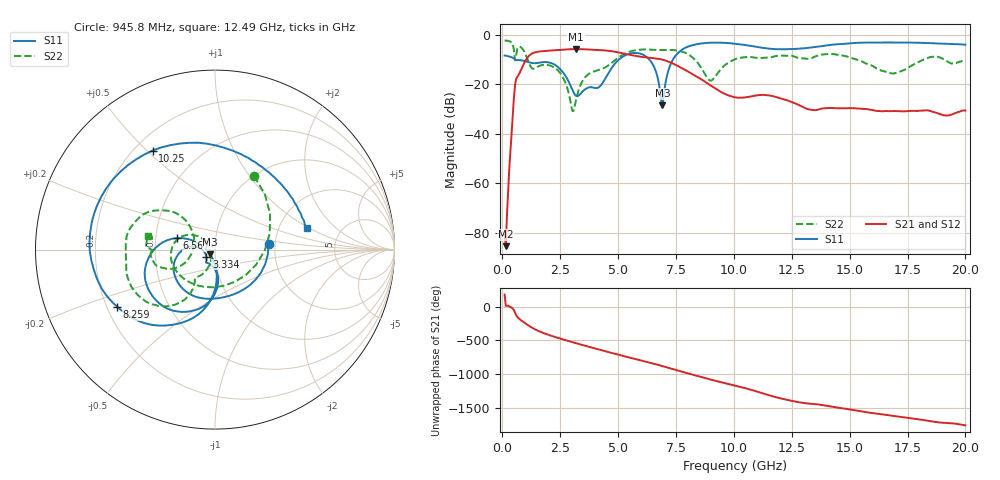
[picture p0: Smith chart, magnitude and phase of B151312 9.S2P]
!  2-Port S-parameters saved by WinCal
! VAR MeasName=S-Parameters (CALIBRATED_DATA) read from VNA (N5244A)
! VAR MeasDate=12/8/2015 5:44:21 PM
! VAR NAME=B151312 9
! VAR FILENAME=B151312 9.S2P
! VAR DATE=12/8/2015 5:44:21 PM
! VAR PHYS_PORTS=1,2
# Hz S DB R 50
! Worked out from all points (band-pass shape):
!   401 points, 100 MHz to 20 GHz, reference 50 ohm
!   highest |S21| = -5.69 dB at 3.184 GHz (marker M1); lowest = -85.4 dB at 149.8 MHz (marker M2)
!   |S21| within 3 dB of the highest: 1.126 GHz to 5.892 GHz (4.766 GHz wide, 136 % of centre)
!   lowest |S11| = -28.5 dB at 6.916 GHz (marker M3), VSWR 1.08, Z = 47.3 - j2.52 ohm
!   |S11| at or under -10 dB: 561.9 MHz to 5.026 GHz (4.464 GHz wide, 160 % of centre); 6.357 GHz to 7.366 GHz (1.009 GHz wide, 14.7 % of centre)
!   |S22| runs from -30.8 to -2.2 dB; largest |S21 - S12| = 0.0016
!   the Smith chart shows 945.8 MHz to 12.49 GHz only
!   S11 on the Smith chart (normalised r, x): 945.8 MHz: 1.84, +0.13; 3.334 GHz: 0.91, -0.07; 6.567 GHz: 0.65, +0.09; 8.259 GHz: 0.24, -0.26; 10.25 GHz: 0.27, +0.52; 12.49 GHz: 2.85, +0.94
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1e8  -8.29 164.7  -79.95 179.5  -91.82 75.4  -2.19 169.3
1.4975e8  -8.36 157.0  -85.43 16.8  -78.04 112.2  -2.22 163.9
5.4775e8  -9.94 89.4  -20.35 -86.6  -20.35 -86.6  -10.27 112.7
9.4575e8  -10.45 6.3  -11.34 123.7  -11.34 123.7  -6.67 62.0
1.64225e9  -11.11 -100.9  -6.62 -13.5  -6.62 -13.5  -12.36 -141.7
2.33875e9  -12.44 -162.1  -6.11 -97.1  -6.11 -97.1  -13.74 160.5
3.1845e9  -24.60 -163.6  -5.69 177.1  -5.70 177.1  -26.26 -114.4
3.33375e9  -24.21 -141.4  -5.71 162.5  -5.71 162.5  -21.33 -109.9
3.43325e9  -23.20 -132.3  -5.74 153.0  -5.74 153.0  -19.17 -111.7
4.92575e9  -10.90 -95.0  -6.86 13.9  -6.86 13.8  -9.75 -121.1
6.5675e9  -13.16 163.0  -9.39 -128.8  -9.38 -128.9  -6.00 -170.7
6.7665e9  -19.77 159.2  -9.64 -148.3  -9.65 -148.2  -6.05 -174.7
6.91575e9  -28.49 -135.1  -9.94 -163.3  -9.96 -163.3  -6.07 -177.5
7.41325e9  -9.28 -101.0  -11.73 146.3  -11.72 146.2  -6.09 169.8
8.259e9  -4.00 -149.7  -16.04 66.1  -16.00 65.9  -9.45 140.1
9.00525e9  -3.09 176.8  -20.44 -3.0  -20.44 -3.5  -18.41 172.0
1.005e10  -3.51 131.1  -25.20 -92.4  -25.24 -92.6  -9.76 -162.7
1.0249e10  -3.72 122.1  -25.37 -109.0  -25.43 -109.2  -9.24 -166.6
1.248775e10  -5.62 13.2  -27.08 41.9  -27.10 42.4  -8.40 168.1
1.338325e10  -5.04 -26.1  -30.33 -3.8  -30.29 -3.3  -9.25 172.1
1.67165e10  -3.03 -113.7  -30.79 -172.8  -30.60 -173.0  -15.33 155.7
2e10  -3.90 -150.1  -30.55 35.8  -30.54 34.8  -10.33 150.1
